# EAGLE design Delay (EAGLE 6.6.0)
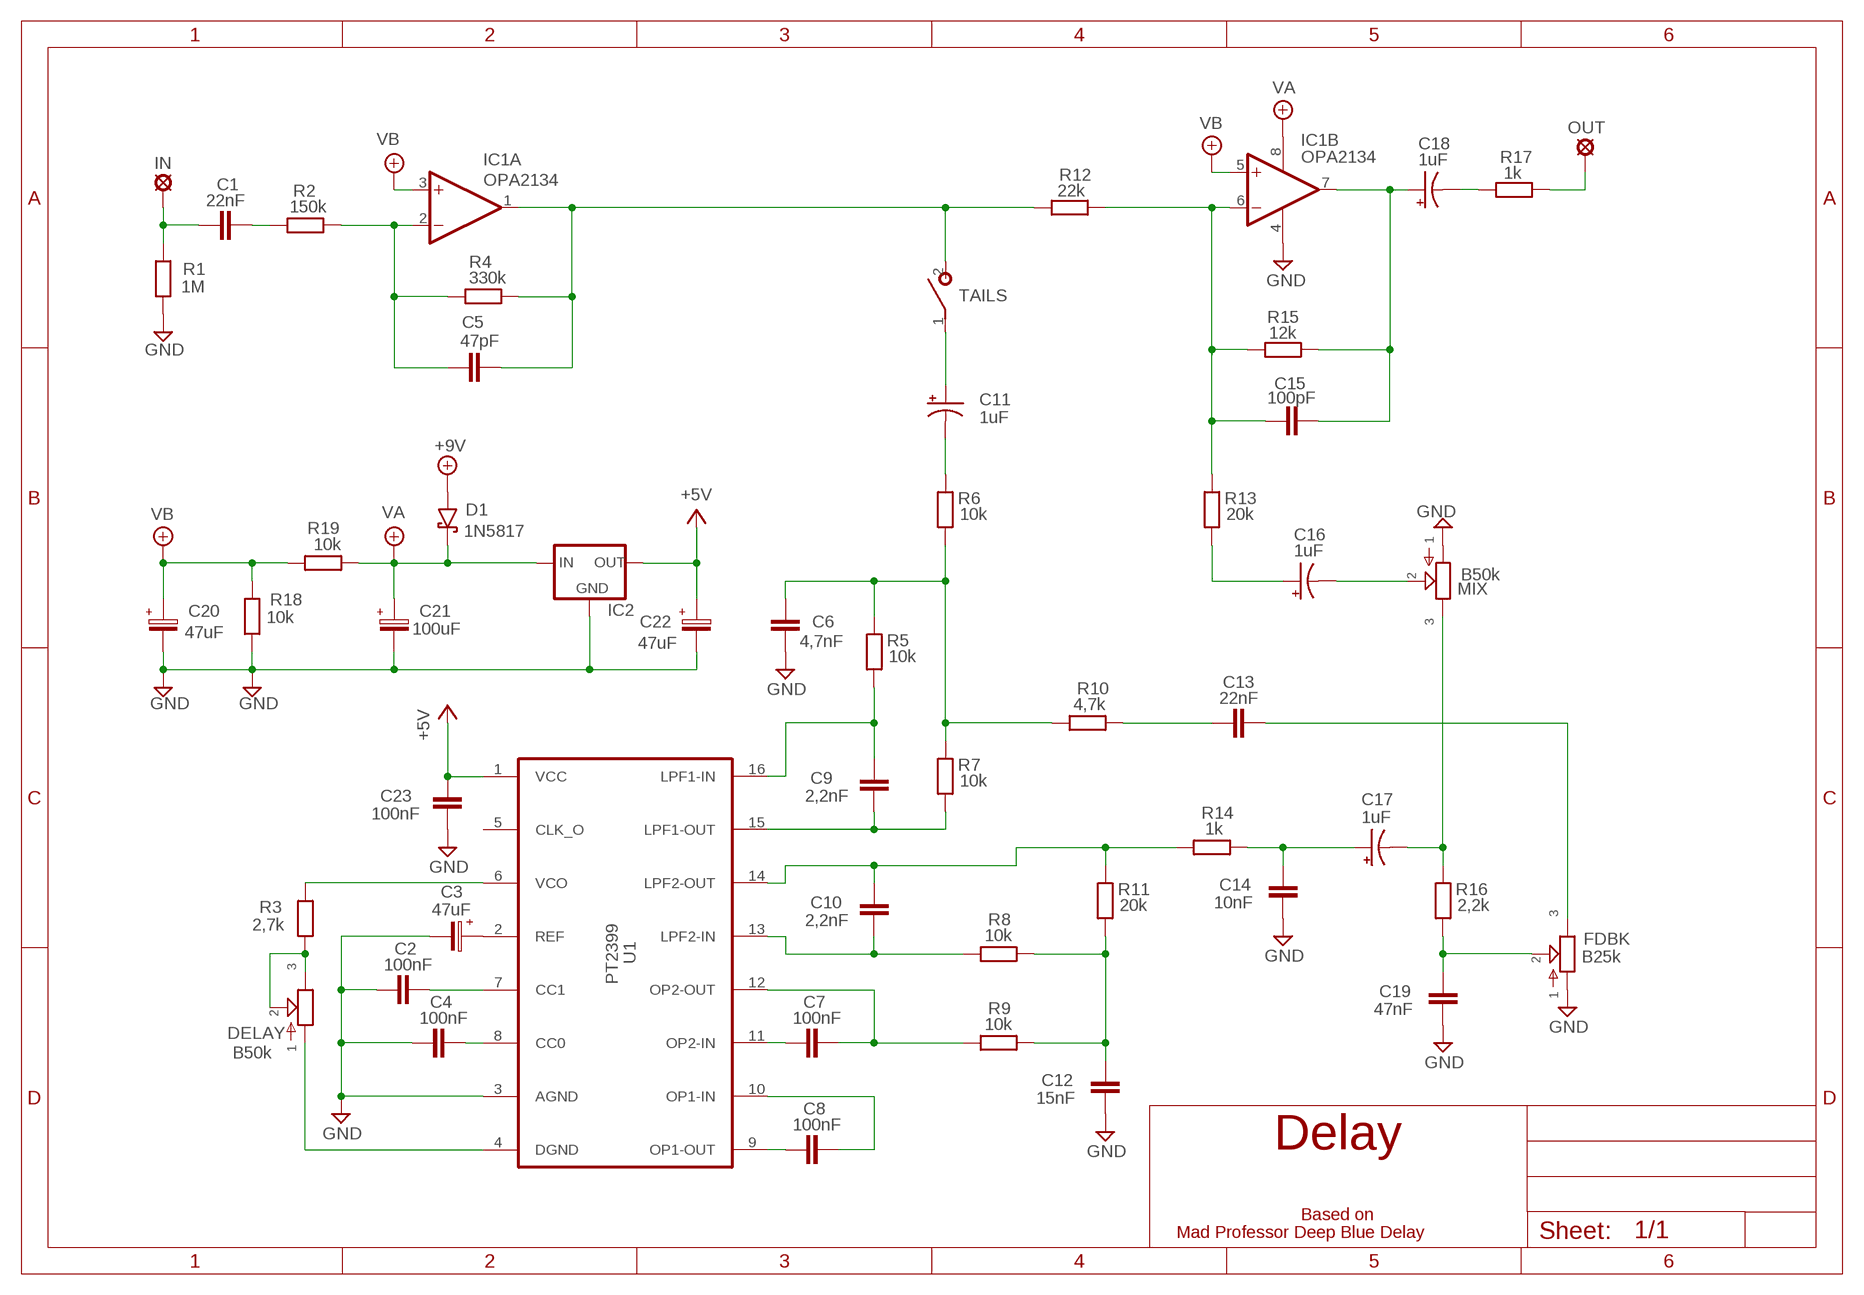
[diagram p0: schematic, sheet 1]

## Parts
+9V  +9V  +9V(T)1  [ROUND]
C1  22nF  22NF-82NF"  [4,5MM]
C2  100nF  050X030_0251  [050X030_025]
C3  47uF  063-EU  [063_025]
C4  100nF  050X030_0251  [050X030_025]
C5  47pF  050X030_0251  [050X030_025]
C6  4,7nF  1NF-15NF  [3,5MM]
C7  100nF  050X030_0251  [050X030_025]
C8  100nF  050X030_0251  [050X030_025]
C9  2,2nF  1NF-15NF  [3,5MM]
C10  2,2nF  1NF-15NF  [3,5MM]
C11  1uF  044A1  [044A]
C12  15nF  1NF-15NF  [3,5MM]
C13  22nF  22NF-82NF"  [4,5MM]
C14  10nF  1NF-15NF  [3,5MM]
C15  100pF  050X030_0251  [050X030_025]
C16  1uF  044A1  [044A]
C17  1uF  044A1  [044A]
C18  1uF  044A1  [044A]
C19  47nF  22NF-82NF"  [4,5MM]
C20  47uF  063-EU  [063_025]
C21  100uF  063-EU  [063_025]
C22  47uF  063-EU  [063_025]
C23  100nF  050X030_0251  [050X030_025]
D1  1N5817  [DO41-3]
DELAY  B50k  POT-EU16MM  [16MM]
FDBK  B25k  POT-EU16MM  [16MM]
GND  GND  GND(T)1  [ROUND]
GND9  GND  GND(T)1  [ROUND]
IC1  OPA2134  TL072P  [DIL08]
IC2  78LXX  [78LXX]
IN  MCS10B  [MCS10B]
MIX  B50k  POT-EU16MM  [16MM]
OUT  MCS10B  [MCS10B]
R1  1M  6MM-EU3  [R0207/3]
R2  150k  6MM-EU3  [R0207/3]
R3  2,7k  6MM-EU3  [R0207/3]
R4  330k  6MM-EU3  [R0207/3]
R5  10k  6MM-EU3  [R0207/3]
R6  10k  6MM-EU3  [R0207/3]
R7  10k  6MM-EU3  [R0207/3]
R8  10k  6MM-EU3  [R0207/3]
R9  10k  6MM-EU3  [R0207/3]
R10  4,7k  6MM-EU3  [R0207/3]
R11  20k  6MM-EU3  [R0207/3]
R12  22k  6MM-EU3  [R0207/3]
R13  20k  6MM-EU3  [R0207/3]
R14  1k  6MM-EU3  [R0207/3]
R15  12k  6MM-EU3  [R0207/3]
R16  2,2k  6MM-EU3  [R0207/3]
R17  1k  6MM-EU3  [R0207/3]
R18  10k  6MM-EU3  [R0207/3]
R19  10k  6MM-EU3  [R0207/3]
TAILS  SPST  [SPST]
U1  PT2399  [DIL16]

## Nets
+5V: C22.+ C23.2 IC2.OUT U1.1(VCC)
+9V: +9V.1(+9V) D1.A
GND: C2.1 C3.- C4.1 C6.1 C12.1 C14.1 C19.1 C20.- C21.- C22.- C23.1 FDBK.1 GND9.1(GND) GND.1(GND) IC1.4(P:V-) IC2.GND MIX.1 R1.1 R18.2 U1.3(AGND)
MIC: C17.2(-) MIX.3 R16.2
N$1: DELAY.2 DELAY.3 R3.1
N$2: R3.2 U1.6(VCO)
N$3: C11.2(-) R6.2
N$4: DELAY.1 U1.4(DGND)
N$5: C4.2 U1.8(CC0)
N$6: C2.2 U1.7(CC1)
N$7: C3.+ U1.2(REF)
N$8: C16.1(+) R13.1
N$9: C1.1 IN.MP R1.2
N$10: C8.2 U1.10(OP1-IN)
N$11: C9.2 R5.1 U1.16(LPF1-IN)
N$12: C9.1 R7.1 U1.15(LPF1-OUT)
N$13: C10.2 R11.2 R14.2 U1.14(LPF2-OUT)
N$14: C1.2 R2.1
N$15: C10.1 R8.2 U1.13(LPF2-IN)
N$16: C5.1 IC1.2(A:-IN) R2.2 R4.1
N$17: C8.1 U1.9(OP1-OUT)
N$18: C7.1 U1.11(OP2-IN)
N$19: C5.2 IC1.1(A:OUT) R4.2 R12.1 TAILS.2(S)
N$20: C18.2(-) R17.1
N$21: C15.1 IC1.6(B:-IN) R12.2 R13.2 R15.1
N$22: C15.2 C18.1(+) IC1.7(B:OUT) R15.2
N$23: OUT.MP R17.2
N$24: C7.2 R9.2 U1.12(OP2-OUT)
N$25: C12.2 R8.1 R9.1 R11.1
N$26: C14.2 C17.1(+) R14.1
N$27: C6.2 R5.2 R6.1 R7.2 R10.2
N$28: C19.2 FDBK.2 R16.1
N$29: C13.1 R10.1
N$30: C13.2 FDBK.3
N$31: C11.1(+) TAILS.1(P)
N$34: C16.2(-) MIX.2
VA: C21.+ D1.C IC1.8(P:V+) IC2.IN R19.1
VB: C20.+ IC1.3(A:+IN) IC1.5(B:+IN) R18.1 R19.2
Unconnected: U1.5(CLK_O)

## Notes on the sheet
- Based on
- Mad Professor Deep Blue Delay

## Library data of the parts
+9V = gm-supply:+9V(T): +9V Voltage Supply
C1 C13 C19 = Mylar Kondensaattorit:22NF-82NF: 22nF-82nF
C2 C4 C5 C7 C8 C15 C23 = Keraamiset kondensaattorit:050X030_025: 47 - 120pF
C3 C20-C22 = Elektrolyytit:063-EU
C6 C9 C10 C12 C14 = Mylar Kondensaattorit:1NF-15NF: 1nF-15nF
C11 C16-C18 = Tantaalit:044A: .1 - 1.5µF
D1 = Diodit:1N5817
DELAY FDBK MIX = gm-pots:POT-EU
GND GND9 = gm-supply:GND(T): Ground
IC1 = Operaatiovahvistimet:TL072: OP AMP
IC2 = v-reg:78LXX: VOLTAGE REGULATOR
IN OUT = Padit:MCS10B: SOLDER PAD
R1-R19 = Vastukset:6MM-EU: 6mm Resistors (European schematic symbol)
TAILS = Kytkimet:SPST
U1 = princeton-tech:PT2399: Echo Processor IC

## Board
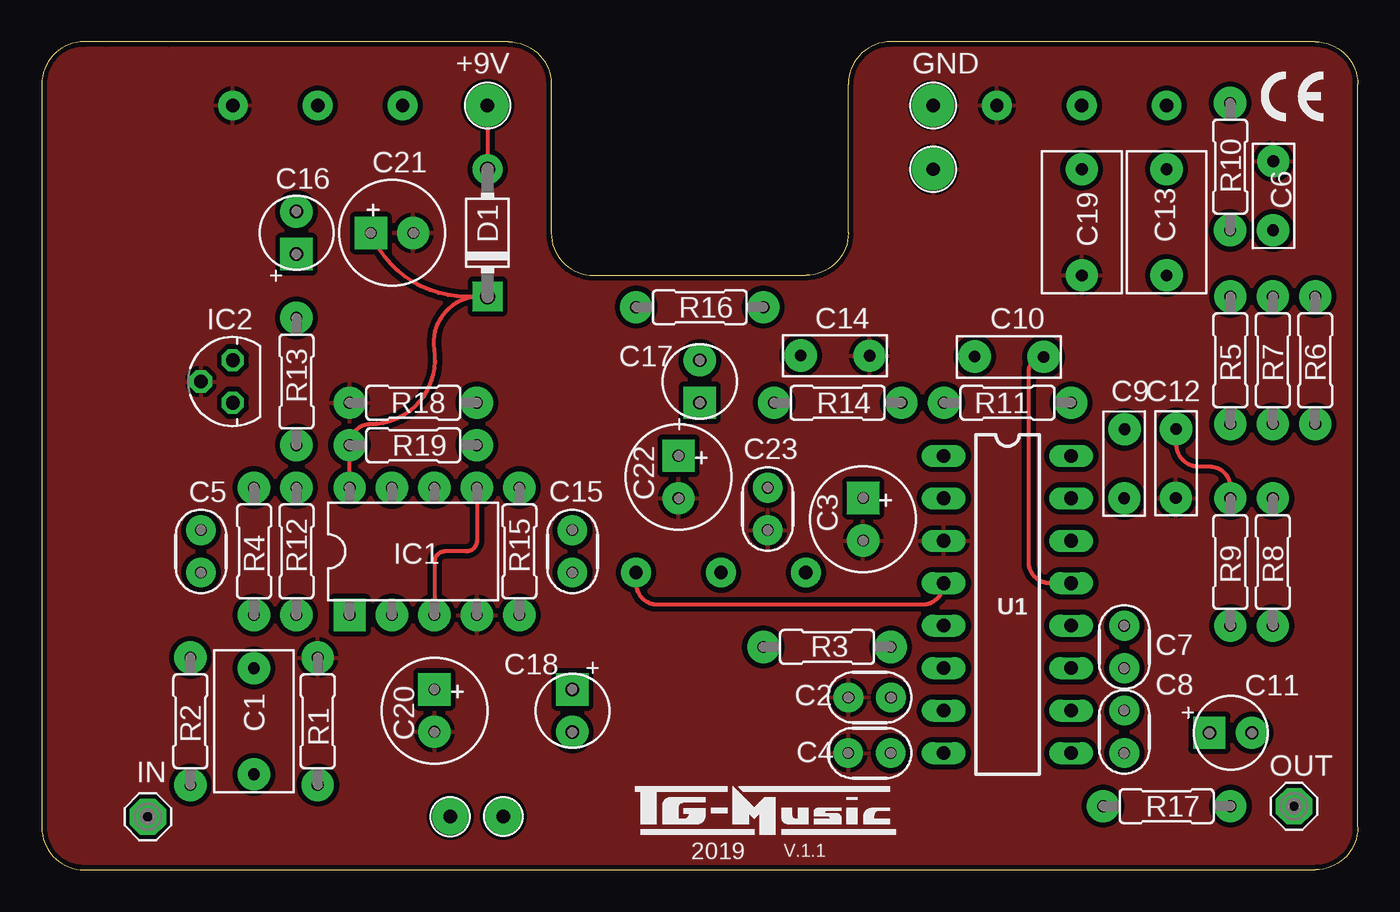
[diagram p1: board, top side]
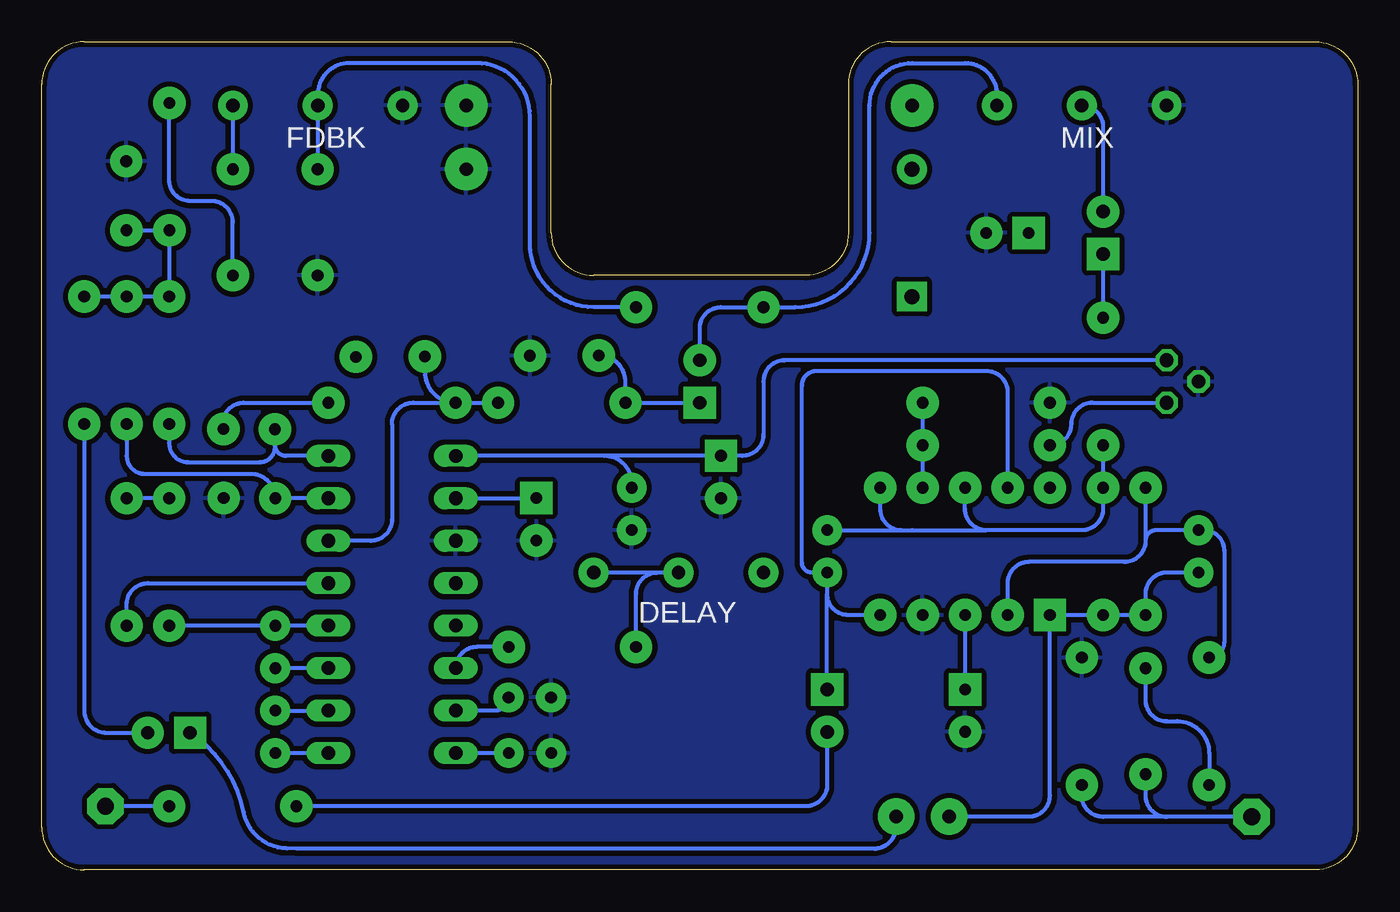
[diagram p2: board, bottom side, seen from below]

Size 78.74 x 49.53 mm. Coordinates in mm from the lower left corner, seen from the top.
Outline: 7.62,49.53 3.81,49.53
Outline: 78.74,2.54 78.74,46.99 arc90 76.2,49.53 50.8,49.53 arc90 48.26,46.99 48.26,38.1 arc-90 45.72,35.56 33.02,35.56 arc-90 30.48,38.1 30.48,46.99 arc90 27.94,49.53 2.54,49.53 arc90 0,46.99 0,2.54 arc90 2.54,0 76.2,0 arc90 78.74,2.54
Copper layers (1*16): Top 0.035mm / dielectric 1.5mm / Bottom 0.035mm
Design rules "ITEADstudio": minimum track width 10mil, minimum drill 12mil, track to track 12mil, track to pad 12mil, pad to pad 12mil, via to via 12mil, smd to smd 0mil, copper to edge 12mil, drill to drill 12mil, minimum pad ring 10mil, minimum via ring 6mil, stop-mask expansion 4mil, vias tented up to drill 100mil, thermal gap 10mil

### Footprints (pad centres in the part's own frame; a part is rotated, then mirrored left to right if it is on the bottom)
ROUND = drill 0.8 pad 2.54: 1 0,0
4,5MM = drill 0.7 pad 1.93: 1 -3.175,0; 2 3.175,0
050X030_025 = drill 0.7 pad 1.778: 1 -1.27,0; 2 1.27,0
063_025 = drill 0.7 pad 1.93 square: + -1.27,0 | drill 0.7 pad 1.93: - 1.27,0
3,5MM = drill 0.7 pad 1.93: 1 -1.905,0; 2 2.221,-0.016
044A = drill 0.8 pad 1.93 square: 1 -1.27,0 | drill 0.8 pad 1.93: 2 1.27,0
DO41-3 = drill 0.9 pad 1.778: A 3.81,0 | drill 0.9 pad 1.778 square: C -3.81,0
16MM = drill 0.8 pad 1.778: 1 5.08,0; 2 0,0; 3 -5.08,0
DIL08 = drill 0.7 pad 1.93 square: 1 -3.81,-3.81 | drill 0.7 pad 1.93: 2 -1.27,-3.81; 3 1.27,-3.81; 4 3.81,-3.81; 5 3.81,3.81; 6 1.27,3.81; 7 -1.27,3.81; 8 -3.81,3.81
78LXX = drill 0.813 octagon: GND 0,1.905; IN -1.27,0; OUT 1.27,0
MCS10B = drill 1.016 pad 2.159 octagon: MP 0,0
R0207/3 = drill 0.7 pad 1.93: 1 -3.81,0; 2 3.81,0
SPST = drill 0.8 pad 2.184: 1 -1.27,0; 2 1.905,0
DIL16 = drill 0.813 long: 1 -8.89,-3.81; 2 -6.35,-3.81; 3 -3.81,-3.81; 4 -1.27,-3.81; 5 1.27,-3.81; 6 3.81,-3.81; 7 6.35,-3.81; 8 8.89,-3.81; 9 8.89,3.81; 10 6.35,3.81; 11 3.81,3.81; 12 1.27,3.81; 13 -1.27,3.81; 14 -3.81,3.81; 15 -6.35,3.81; 16 -8.89,3.81

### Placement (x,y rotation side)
+9V  26.67,45.72 0 top
C1  12.7,8.89 90 top
C2  49.54,10.31 0 top
C3  49.14,20.97 270 top
C4  49.53,6.99 0 top
C5  9.53,19.05 270 top
C6  73.69,40.48 270 top
C7  64.77,13.34 90 top
C8  64.77,8.26 90 top
C9  64.77,24.13 90 top
C10  58.04,30.68 180 top
C11  71.14,8.2 0 top
C12  67.86,24.15 90 top
C13  67.31,38.73 90 top
C14  47.62,30.75 180 top
C15  31.75,19.05 270 top
C16  15.24,38.1 90 top
C17  39.37,29.21 90 top
C18  31.75,9.53 270 top
C19  62.23,38.73 90 top
C20  23.5,9.53 270 top
C21  20.95,38.1 0 top
C22  38.1,23.5 270 top
C23  43.44,21.59 90 top
D1  26.67,38.1 90 top
DELAY  40.64,17.78 0 bottom
FDBK  62.23,45.72 0 bottom
GND  53.34,45.72 0 top
GND9  53.34,41.91 0 top
IC1  22.23,19.05 0 top
IC2  11.43,29.21 90 top
IN  6.35,3.17 0 top
MIX  16.51,45.72 0 bottom
OUT  74.93,3.81 0 top
R1  16.51,8.89 270 top
R2  8.89,8.89 90 top
R3  46.99,13.34 0 top
R4  12.7,19.05 270 top
R5  71.12,30.48 90 top
R6  76.2,30.48 270 top
R7  73.66,30.48 90 top
R8  73.66,18.41 270 top
R9  71.12,18.41 270 top
R10  71.11,42.06 270 top
R11  57.78,27.94 180 top
R12  15.24,19.05 90 top
R13  15.24,29.21 270 top
R14  47.62,27.94 0 top
R15  28.57,19.05 270 top
R16  39.37,33.66 180 top
R17  67.31,3.81 0 top
R18  22.23,27.94 180 top
R19  22.23,25.4 0 top
TAILS  26.35,3.19 180 top
U1  57.78,15.88 270 top

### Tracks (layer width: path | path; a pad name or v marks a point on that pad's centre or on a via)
+5V
  Bottom 0.254: 45.09,24.77 C22.+ 36.83,24.77 arc-90 35.56,26.04 35.56,29.21 arc90 34.29,30.48 IC2.OUT | 45.09,24.77 U1.1 | C23.2 43.44,23.12 arc-90 45.09,24.77
+9V
  Top 0.254: +9V.1 D1.A
GND
  pour Bottom: 0,2.54 0,46.99 arc-90 2.54,49.53 27.94,49.53 arc-90 30.48,46.99 30.48,38.1 arc90 33.02,35.56 45.72,35.56 arc90 48.26,38.1 48.26,46.99 arc-90 50.8,49.53 76.2,49.53 arc-90 78.74,46.99 78.74,2.54 arc-90 76.2,0 2.54,0 arc-90
  pour Top: 0,2.54 0,46.99 arc-90 2.54,49.53 27.94,49.53 arc-90 30.48,46.99 30.48,38.1 arc90 33.02,35.56 45.72,35.56 arc90 48.26,38.1 48.26,46.99 arc-90 50.8,49.53 76.2,49.53 arc-90 78.74,46.99 78.74,2.54 arc-90 76.2,0 2.54,0 arc-90
MIC
  Bottom 0.254: MIX.3 21.59,46.35 arc-90 23.5,48.26 26.67,48.26 arc-90 29.21,45.72 29.21,38.1 arc90 33.66,33.66 R16.2 38.1,33.66 arc-90 39.37,32.38 C17.2
N$1
  Bottom 0.254: DELAY.2 41.91,17.78 | 41.91,17.78 DELAY.3 | R3.1 43.18,16.51 arc90 41.91,17.78
N$2
  Bottom 0.254: R3.2 52.7,13.34 arc-90 U1.6
N$3
  Bottom 0.254: R6.2 76.2,9.53 arc-90 74.88,8.2 C11.2
N$4
  Top 0.254: DELAY.1 35.56,17.14 arc90 36.83,15.88 52.7,15.88 arc90 U1.4
N$5
  Bottom 0.254: C4.2 U1.8
N$6
  Bottom 0.254: C2.2 arc90 51.6,9.53 U1.7
N$7
  Bottom 0.254: C3.+ U1.2
N$8
  Bottom 0.254: C16.1 R13.1
N$9
  Bottom 0.254: IN.MP 11.43,3.17 | 11.43,3.17 15.24,3.17 arc90 16.51,4.45 R1.2 | C1.1 12.7,4.45 arc-90 11.43,3.17
N$10
  Bottom 0.254: C8.2 U1.10
N$11
  Bottom 0.254: R5.1 71.12,25.52 arc-90 69.99,24.39 65.69,24.39 arc-90 64.78,25.3 64.78,25.4 | 64.78,25.4 C9.2 arc-90 C9.2 | U1.16 64.15,24.77 arc90 64.78,25.4
N$12
  Bottom 0.254: U1.15 C9.1 arc-90 66.23,23.69 72.58,23.69 arc90 73.66,24.77 R7.1
N$13
  Bottom 0.254: U1.14 59.05,19.68 arc-90 57.78,20.95 57.78,26.67 arc90 56.52,27.94 R11.2 | R11.2 R14.2 | C10.2 55.81,29.78 arc-90 R11.2
N$14
  Bottom 0.254: C1.2 12.7,10.16 arc-90 11.43,8.89 10.79,8.89 arc90 8.89,6.99 R2.1
N$15
  Top 0.254: U1.13 60.33,17.14 arc-90 59.05,18.41 59.05,29.8 arc-90 C10.1
  Bottom 0.254: R8.2 73.66,15.88 arc90 72.39,17.14 U1.13
N$16
  Bottom 0.254: R4.1 12.7,19.68 | 12.7,19.68 arc90 13.97,18.41 19.68,18.41 arc-90 20.95,17.14 IC1.2 | 12.7,19.68 arc90 12.06,20.32 C5.1 9.21,20.32 arc90 8,19.11 8,13.59 arc90 R2.2
N$17
  Bottom 0.254: U1.9 C8.1
N$18
  Bottom 0.254: U1.11 C7.1
N$19
  Bottom 0.254: C5.2 11.43,17.78 arc-90 12.7,16.51 R4.2 R12.1 IC1.1 18.41,4.45 arc90 19.66,3.19 TAILS.2
N$20
  Bottom 0.254: C18.2 31.75,5.08 arc90 33.02,3.81 R17.1
N$21
  Bottom 0.254: R13.2 R12.2 15.24,21.59 arc90 16.51,20.32 22.23,20.32 | 22.23,20.32 arc90 23.5,21.59 IC1.6 | R15.1 28.57,21.59 arc-90 27.3,20.32 26.67,20.32 | 26.67,20.32 22.23,20.32 | C15.1 26.67,20.32
N$22
  Bottom 0.254: 31.75,16.51 C15.2 32.66,17.78 arc90 33.25,18.36 33.25,28.98 arc90 32.38,29.84 22.23,29.84 arc90 20.95,28.57 IC1.7 | R15.2 30.48,15.24 arc90 31.75,16.51 | C18.1 31.75,16.51
N$23
  Bottom 0.254: R17.2 OUT.MP
N$24
  Bottom 0.254: U1.12 C7.2 R9.2
N$25
  Top 0.254: C12.2 67.88,25.47 arc90 69.22,24.13 69.85,24.13 arc-90 71.12,22.86 R9.1
  Bottom 0.254: R9.1 R8.1 | C12.2 67.88,26.74 arc90 66.67,27.94 R11.1
N$26
  Bottom 0.254: C17.1 R14.1 43.81,29.18 arc-90 C14.2
N$27
  Bottom 0.254: R6.1 R7.2 R5.2 arc-90 71.11,34.3 R10.2 arc-90 R10.2 C6.2
N$28
  Bottom 0.254: R16.1 45.72,33.66 arc90 49.53,37.47 49.53,45.09 arc-90 52.7,48.26 60.33,48.26 arc-90 62.23,46.35 FDBK.2 C19.2
N$29
  Bottom 0.254: C13.1 67.31,38.73 arc-90 68.58,40.01 69.85,40.01 arc90 71.12,41.27 R10.1 arc90 R10.1
N$30
  Bottom 0.254: FDBK.3 C13.2
N$31
  Bottom 0.254: TAILS.1 arc90 27.6,3.17 27.6,2.63 arc90 28.96,1.27 63.5,1.27 64.09,1.29 arc77 66.66,3.45 arc-45 C11.1
N$34
  Bottom 0.254: MIX.2 arc90 15.24,44.45 C16.2
VA
  Top 0.254: IC1.8 R19.1 arc-90 19.68,26.67 arc99 23.5,31.11 arc-108 D1.C 25.4,34.29 arc-67 C21.+
  Bottom 0.254: R19.1 arc-90 17.14,26.67 arc90 15.88,27.94 IC2.IN
VB
  Top 0.254: IC1.5 26.04,19.68 arc-90 25.4,19.05 24.13,19.05 arc90 23.5,18.41 IC1.3
  Bottom 0.254: R18.1 R19.2 IC1.5 | IC1.3 C20.+

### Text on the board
tNames: 2019 | V.1.1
